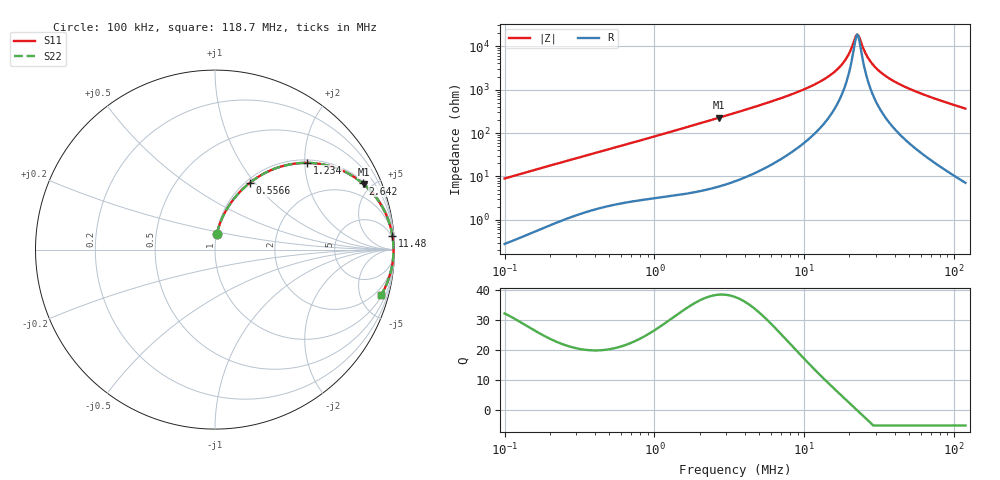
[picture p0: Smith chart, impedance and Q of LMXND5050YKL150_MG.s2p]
! LMXND5050YKL150_MG  S-PARAMETER MODEL  ( General Type )
! Model Generated by TAIYO YUDEN Corporation (https://www.yuden.co.jp/en/)
! Version 1.0
! TAIYO YUDEN Control No. 191023NI43SB-FBB
! Copyright(c) 2019 TAIYO YUDEN CO.,LTD. All Rights Reserved.
! Product Description (link to TY-COMPAS)
! https://ds.yuden.co.jp/TYCOMPAS/or/detail?pn=LMXND5050YKL150MMG&u=M
! Products Name : Inductors
! Characteristics :
!  Inductance : 15 uH , SRF(min) : 13 MHz , DC Resistance(max) : 0.104 Ohm
!  Rated Current : Saturation :2000 mA , Temp Rise : 1800 mA (40 degC)
!  Case Size : 4.9 x 4.9 / 0.193 x 0.193 [mm/inch] , Thickness : 4 / 0.157 [mm/inch]
!  (Conditions: Temperature = 25 degC , DC Bias Current/Voltage = 0A / 0V)
! External Node Assignments :
!  1  o---GGG---o  2
! GND o---------o GND
! Frequency Range : 0.1MHz  -  118.695536MHz  [ 402 STEP ]
# MHz S RI R 50
! Freq[MHz].  S11 Real  S11 Imag  S21 Real  S21 Imag  S12 Real  S12 Imag  S22 Real  S22 Imag
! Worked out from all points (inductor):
!   401 points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, 100 kHz to 118.7 MHz, reference 50 ohm
!   read as one part in series: L = 14.2 uH near 103.6 kHz
!   highest Q = 38.4 at 2.689 MHz (marker M1), where L = 13.3 uH
!   self-resonance near 22.49 MHz
!   S11 on the Smith chart (normalised r, x): 100 kHz: 1.01, +0.18; 556.6 kHz: 1.05, +0.95; 1.234 MHz: 1.07, +2.05; 2.642 MHz: 1.12, +4.41; 11.48 MHz: 3, +25; 118.7 MHz: 1.14, -7.32
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0.1  0.0107 0.0885  0.9893 -0.0885  0.9893 -0.0885  0.0107 0.0885
0.327316  0.0858 0.2565  0.9142 -0.2565  0.9142 -0.2565  0.0858 0.2565
0.556609  0.1943 0.3723  0.8057 -0.3723  0.8057 -0.3723  0.1943 0.3723
1.07136  0.446 0.4792  0.554 -0.4792  0.554 -0.4792  0.446 0.4792
1.23431  0.5132 0.4832  0.4868 -0.4832  0.4868 -0.4832  0.5132 0.4832
2.641958  0.8234 0.3685  0.1766 -0.3685  0.1766 -0.3685  0.8234 0.3685
2.689131  0.8285 0.3641  0.1715 -0.3641  0.1715 -0.3641  0.8285 0.3641
3.445222  0.8877 0.3027  0.1123 -0.3027  0.1123 -0.3027  0.8877 0.3027
6.870282  0.9691 0.1545  0.0309 -0.1545  0.0309 -0.1545  0.9691 0.1545
11.27678  0.988 0.0794  0.012 -0.0794  0.012 -0.0794  0.988 0.0794
11.47813  0.9884 0.0771  0.0116 -0.0771  0.0116 -0.0771  0.9884 0.0771
14.70538  0.9923 0.0469  0.00767 -0.0469  0.00767 -0.0469  0.9923 0.0469
17.55242  0.9939 0.027  0.00612 -0.027  0.00612 -0.027  0.9939 0.027
19.51882  0.9944 0.0155  0.0056 -0.0155  0.0056 -0.0155  0.9944 0.0155
21.70552  0.9947 0.00413  0.00535 -0.00413  0.00535 -0.00413  0.9947 0.00413
22.48756  0.9947 0.000358  0.00533 -0.000358  0.00533 -0.000358  0.9947 0.000358
23.29778  0.9947 -0.00342  0.00533 0.00342  0.00533 0.00342  0.9947 -0.00342
25.45335  0.9945 -0.0129  0.00547 0.0129  0.00547 0.0129  0.9945 -0.0129
27.80836  0.9942 -0.0224  0.0058 0.0224  0.0058 0.0224  0.9942 -0.0224
36.91074  0.9917 -0.0545  0.00826 0.0545  0.00826 0.0545  0.9917 -0.0545
58.47779  0.981 -0.116  0.019 0.116  0.019 0.116  0.981 -0.116
118.6955  0.9263 -0.2517  0.0737 0.2517  0.0737 0.2517  0.9263 -0.2517
